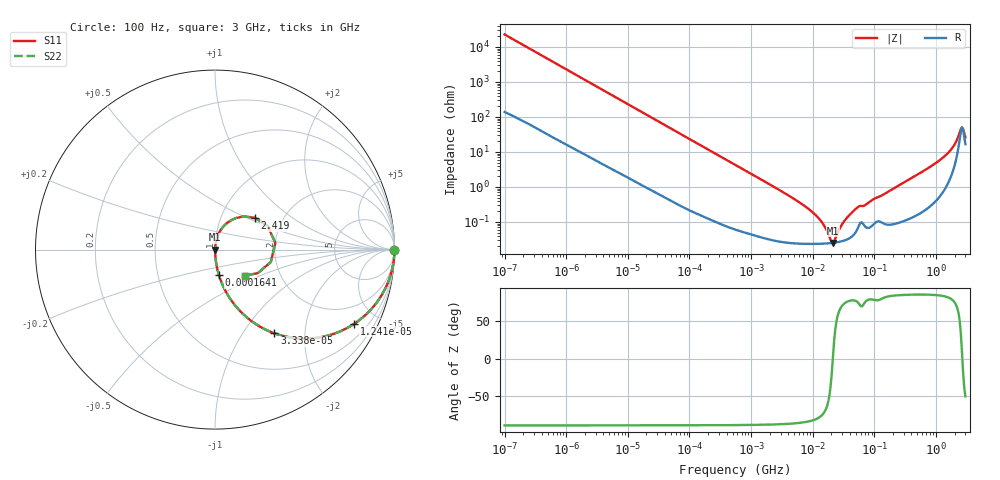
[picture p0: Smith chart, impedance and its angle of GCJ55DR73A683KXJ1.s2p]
!Murata Part Number: GCJ55DR73A683KXJ1
!These Parameters are Measured in Series Mode Connection
!Data Generated on Mar 13, 2026
!  o--ll--o
!Port1  Port2
!  o------o
!Operation Temp=25[degC], DC Bias Voltage=0[V]
!Freq. Start=100[Hz] Stop=3[GHz] 401[Steps]
# Hz S RI R 50
!Freq.(Hz) S11(Real) S11(Imag) S21(Real) S21(Imag) S12(Real) S12(Imag) S22(Real) S22(Imag)
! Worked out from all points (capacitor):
!   401 points, 100 Hz to 3 GHz, reference 50 ohm
!   read as one part in series: C = 69.9 nF near 109 Hz
!   lowest |Z| = 25.4 mohm at 21.25 MHz (marker M1)
!   series resonance near 21.18 MHz, so ESL is about 810 pH
!   S11 on the Smith chart (normalised r, x): 100 Hz: open; 12.4 kHz: 1.03, -3.75; 33.38 kHz: 1.01, -1.40; 164.1 kHz: 1.00, -0.29; 2.419 GHz: 1.44, +0.56; 3 GHz: 1.33, -0.41
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100  1 -0.00439  4.62e-05 0.00439  4.62e-05 0.00439  1 -0.00439
1788  0.9935 -0.077  0.00654 0.077  0.00654 0.077  0.9935 -0.077
5716  0.9411 -0.2316  0.0589 0.2316  0.0589 0.2316  0.9411 -0.2316
12405  0.777 -0.4123  0.223 0.4123  0.223 0.4123  0.777 -0.4123
31977  0.3498 -0.4727  0.6502 0.4727  0.6502 0.4727  0.3498 -0.4727
33383  0.3308 -0.4663  0.6692 0.4663  0.6692 0.4663  0.3308 -0.4663
66468  0.1131 -0.3124  0.8869 0.3124  0.8869 0.3124  0.1131 -0.3124
164120  0.0216 -0.1404  0.9784 0.1404  0.9784 0.1404  0.0216 -0.1404
547723  0.00248 -0.0432  0.9975 0.0432  0.9975 0.0432  0.00248 -0.0432
4141163  0.000283 -0.00558  0.9997 0.00558  0.9997 0.00558  0.000283 -0.00558
9794414  0.00024 -0.00193  0.9998 0.00193  0.9998 0.00193  0.00024 -0.00193
1.382041e7  0.00024 -0.001  0.9998 0.001  0.9998 0.001  0.00024 -0.001
1.950129e7  0.000249 -0.000188  0.9998 0.000188  0.9998 0.000188  0.000249 -0.000188
2.12544e7  0.000253 8.7e-06  0.9997 -8.7e-06  0.9997 -8.7e-06  0.000253 8.7e-06
3.268714e7  0.000297 0.00103  0.9997 -0.00103  0.9997 -0.00103  0.000297 0.00103
5.026954e7  0.000531 0.00234  0.9995 -0.00234  0.9995 -0.00234  0.000531 0.00234
1.751444e8  0.000891 0.00764  0.9991 -0.00764  0.9991 -0.00764  0.000891 0.00764
1.214989e9  0.00984 0.0616  0.9902 -0.0616  0.9902 -0.0616  0.00984 0.0616
1.950712e9  0.053 0.1354  0.947 -0.1354  0.947 -0.1354  0.053 0.1354
2.419119e9  0.222 0.1774  0.778 -0.1774  0.778 -0.1774  0.222 0.1774
2.636591e9  0.3362 0.0375  0.6638 -0.0375  0.6638 -0.0375  0.3362 0.0375
3e9  0.1683 -0.1449  0.8317 0.1449  0.8317 0.1449  0.1683 -0.1449
